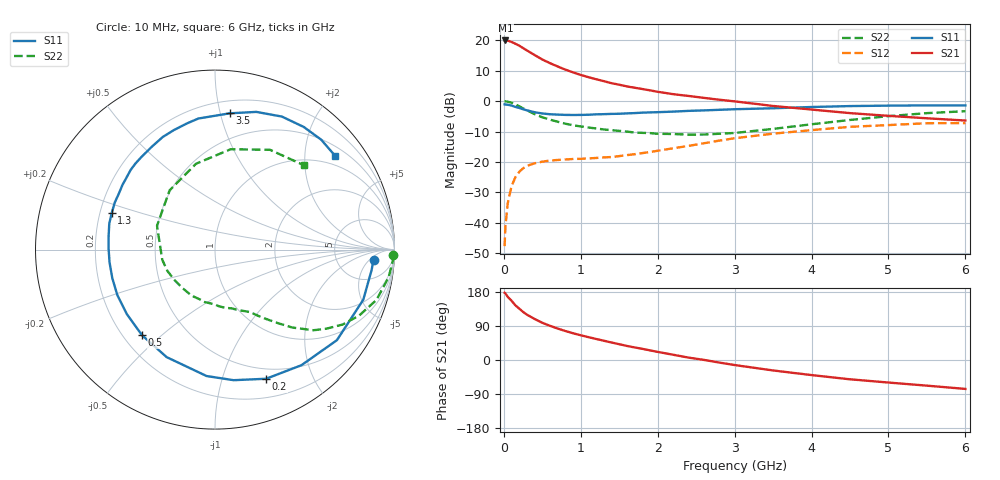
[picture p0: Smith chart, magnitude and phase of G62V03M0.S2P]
! SIEMENS Small Signal Semiconductors
! BFG193
! Si NPN RF Bipolar Junction Transistor in SOT223
! VCE = 2 V  IC = 3 mA
! Common Emitter S-Parameters:  August  1996
# GHz  S  MA  R  50
!  f  S11  S21  S12  S22
! GHz  MAG  ANG  MAG  ANG  MAG  ANG  MAG  ANG
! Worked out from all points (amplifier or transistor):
!   36 points, 10 MHz to 6 GHz, reference 50 ohm
!   highest |S21| = 20.0 dB at 20 MHz (marker M1)
!   |S21| within 3 dB of that: start of sweep to 281.6 MHz
!   unconditionally stable (mu >= 1): 1.27 GHz to 2.696 GHz
!   at 250 MHz: K = 0.24, MSG = 19.8 dB, |S12| = -22.1 dB
!   at 1.4 GHz: K = 1.07, MAG = 10.5 dB, |S12| = -18.4 dB
!   at 6 GHz: K = 0.95, MSG = 0.4 dB, |S12| = -7.2 dB
!   S11 on the Smith chart (normalised r, x): 10 MHz: 13, -7; 200 MHz: 0.39, -1.40; 500 MHz: 0.28, -0.43; 1.3 GHz: 0.25, +0.16; 3.5 GHz: 0.29, +1.07; 6 GHz: 0.73, +2.73
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0.01  0.8857 -3.6  9.961 177.4  0.0041 90.6  0.993 -1.8
0.02  0.8795 -7.7  9.977 175.7  0.0084 85.3  0.9928 -3.6
0.05  0.872 -18.7  9.901 166.8  0.0207 78.4  0.9797 -9.0
0.1  0.8462 -36.6  9.445 156.4  0.0398 71.3  0.9425 -17.3
0.15  0.8043 -53.2  8.793 144.3  0.056 61.6  0.8832 -24.6
0.2  0.7739 -68.4  8.185 135.6  0.0686 55.2  0.8248 -30.4
0.25  0.7349 -81.9  7.479 126.9  0.0784 48.9  0.7608 -35.4
0.3  0.706 -93.8  6.831 119.7  0.086 44.3  0.7093 -39.3
0.4  0.6569 -114.2  5.748 108.3  0.0948 37.3  0.612 -45.2
0.5  0.6268 -130.4  4.842 98.2  0.101 31.9  0.5429 -49.2
0.6  0.6087 -143.7  4.22 90.2  0.1051 29.1  0.4958 -52.4
0.7  0.6003 -155.0  3.722 83.0  0.1076 26.8  0.4578 -55.5
0.9  0.5918 -173.2  2.976 70.6  0.1117 25.0  0.4009 -60.5
1.1  0.5975 172.7  2.48 60.3  0.1142 24.8  0.3683 -67.2
1.3  0.6106 160.3  2.133 50.8  0.1186 25.6  0.3417 -73.7
1.6  0.6292 145.0  1.748 37.1  0.1291 27.3  0.3158 -86.3
2.2  0.6723 121.7  1.304 13.9  0.1675 28.3  0.2877 -117.1
2.8  0.72 102.6  1.056 -6.7  0.224 22.4  0.2906 -155.8
3.5  0.7638 83.8  0.833 -27.6  0.2915 8.1  0.3494 157.6
4.5  0.8296 63.3  0.635 -50.9  0.378 -13.5  0.4901 102.4
5.5  0.8515 46.0  0.522 -67.7  0.4331 -39.9  0.6349 61.1
6  0.8491 38.0  0.48 -76.3  0.4356 -54.5  0.6829 43.5
